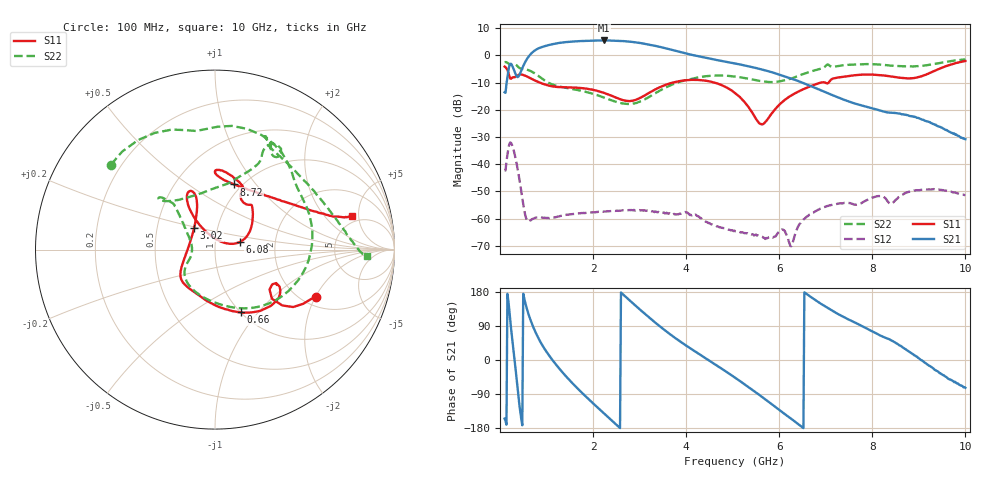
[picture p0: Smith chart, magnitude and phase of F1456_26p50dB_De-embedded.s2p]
! Integrated Device Technology
! Corporate Headquarters
! 6024 Silver Creek Valley Road
! San Jose, CA 95138  USA
! Phone:  1-408-284-8200
! Toll Free:  1-800-223-1366
! Webpage:  http://www.idt.com/
! Timing and RF Division
! 515 Groton Road, Suite 102
! Westford, MA 01886-6024
! Device:  F1456
! Description: 6-bit 0.5 dB Transmit Variable Gain Amplifier
! Frequency:  2100.0 -  2950.00 MHz
! Package:  6x6 mm Thin QFN Plastic Package: 28 pin
! State:  53
! Atten State:  26.5 dB
! Voltage:  +5.00 Volts
! Current:  216.948 mA
! Data:  The device was measured on a the F1455 evaluation board which has
!  individual transmission lines to the RF pins.  Data was collected
!  using a calibrated network analyzer.  The evaluation board was
!  de-embedded using a TRL calibration technique.
!  The reference plane is the edge of the package pin.
!  Pin  1 = CSb
!  Pin  2 = DATA
!  Pin  3 = CLK
!  Pin  4 = RSET
!  Pin  5 = GND
!  Pin  6 = RFIN  = Port 1
!  Pin  7 = GND
!  Pin  8 = NC
!  Pin  9 = NC
!  Pin 10 = NC
!  Pin 11 = NC
!  Pin 12 = NC
!  Pin 13 = NC
!  Pin 14 = /STBY
!  Pin 15 = GND
!  Pin 16 = RFOUT  = Port 2
!  Pin 17 = GND
!  Pin 18 = NC
!  Pin 19 = NC
!  Pin 20 = NC
!  Pin 21 = GND
!  Pin 22 = NC
!  Pin 23 = GND
!  Pin 24 = NC
!  Pin 25 = NC
!  Pin 26 = NC
!  Pin 27 = GND
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# GHz S dB R 50
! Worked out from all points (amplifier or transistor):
!   496 points, 100 MHz to 10 GHz, reference 50 ohm
!   highest |S21| = 5.5 dB at 2.24 GHz (marker M1)
!   |S21| within 3 dB of that: 816.7 MHz to 3.589 GHz (2.772 GHz wide, 126 % of centre)
!   unconditionally stable (mu >= 1): start of sweep to end of sweep
!   at 1.74 GHz: K = 191.76, MAG = 5.8 dB, |S12| = -57.9 dB
!   at 5.06 GHz: K = 965.92, MAG = -2.0 dB, |S12| = -64.6 dB
!   at 10 GHz: K = 696.65, MAG = -21.2 dB, |S12| = -51.3 dB
!   S11 on the Smith chart (normalised r, x): 100 MHz: 2.37, -2.03; 660 MHz: 1.00, -0.82; 3.02 GHz: 0.77, +0.19; 6.08 GHz: 1.31, +0.11; 8.72 GHz: 0.92, +0.78; 10 GHz: 4.20, +4.13
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0.1  -4.12 -24.9  -13.56 -154.8  -42.31 49.9  -2.52 140.8
0.24  -8.56 -31.2  -3.13 81.8  -32.20 -77.2  -3.44 94.5
0.32  -8.00 -29.1  -6.21 -6.3  -36.63 -155.4  -3.23 67.9
0.42  -7.04 -36.6  -7.15 -121.0  -45.75 139.7  -4.66 40.6
0.54  -7.44 -53.5  -2.52 152.8  -58.44 122.4  -5.08 16.4
0.66  -8.46 -67.7  0.47 104.5  -60.59 141.5  -5.76 -11.3
0.84  -9.88 -86.0  2.66 54.3  -59.54 115.7  -7.73 -49.4
1.16  -11.47 -111.8  4.21 -5.2  -59.54 81.5  -10.89 -95.5
1.76  -12.04 -139.0  5.27 -86.3  -57.91 46.6  -13.04 -139.4
2.24  -13.81 -154.4  5.47 -141.6  -57.36 28.0  -15.53 -155.1
2.62  -16.35 179.9  5.28 175.9  -56.94 13.9  -17.64 -170.4
3.02  -15.56 134.4  4.52 131.8  -56.96 -4.0  -16.86 162.1
3.4  -11.97 113.4  3.25 92.3  -57.49 -19.9  -13.32 142.3
4.1  -9.01 112.7  0.26 30.1  -58.56 -53.1  -8.70 133.1
5.06  -13.93 122.9  -3.02 -47.4  -64.64 -104.2  -7.80 137.7
5.62  -25.34 66.6  -5.15 -96.5  -66.51 -165.4  -9.49 122.4
6.08  -16.89 17.1  -7.52 -139.1  -64.00 154.5  -9.30 90.1
6.26  -14.72 21.3  -8.56 -155.3  -70.09 160.2  -8.51 78.9
6.7  -11.15 40.7  -11.44 164.6  -58.03 145.5  -5.82 64.4
8.36  -7.63 88.7  -21.03 55.0  -54.23 61.5  -3.74 62.4
8.72  -8.44 73.8  -21.81 28.5  -50.47 66.7  -4.04 50.2
10  -2.08 13.8  -30.80 -73.4  -51.34 -26.4  -1.46 -2.6
